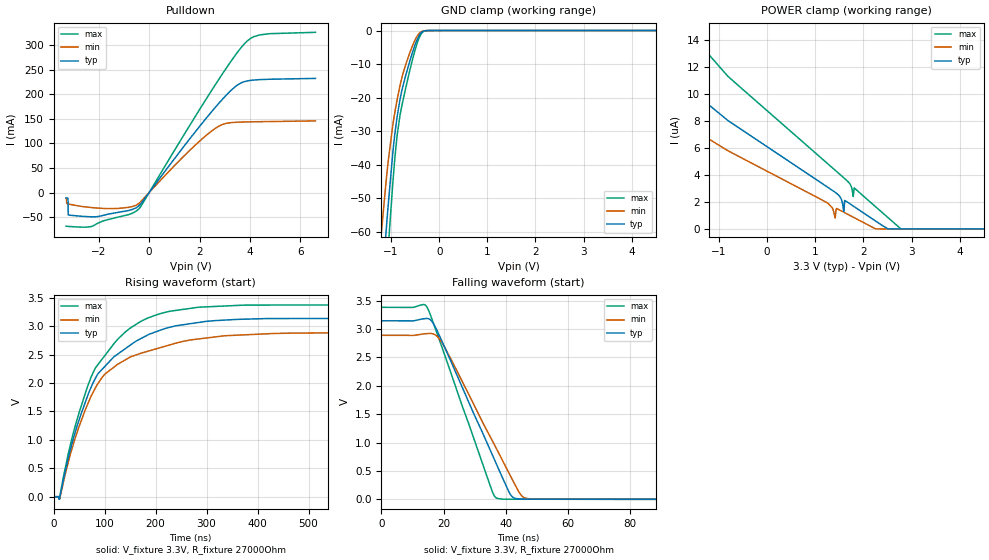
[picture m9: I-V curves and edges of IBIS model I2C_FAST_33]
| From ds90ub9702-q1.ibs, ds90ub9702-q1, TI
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|   I2C_Fast_33 Model
[Model]   I2C_FAST_33
Model_type   I/O_open_drain
Polarity   Non-Inverting
Enable   Active-High
Vinl = 0.99
Vinh = 2.31
Vmeas = 1.65
Vref = 3.3
Cref = 0pF
Rref = 27000
|   typ   min   max
C_comp   1.392003pF   1.392003pF   1.392003pF
[Voltage Range]   3.3   3   3.6
[Temperature Range]   27   105   -40
[Pullup Reference]   3.3   3   3.6
[Pulldown Reference]   -0   0   -0
[Power Clamp Reference]   3.3   3   3.6
[GND Clamp Reference]   0   0   0
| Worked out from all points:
|   slope of the pulldown table from 0 to 0.495 V, typ, clamps not added: 14.5 ohm
|   GND clamp passes 1 mA (typ) near -0.39 V on its own axis
|   falling waveform, V_fixture 3.3V, R_fixture 27000Ohm: 20-80 % time 15.3ns typ, 16.1ns min, 12.9ns max; typ from 3.14 V to 0.002 V
|   rising waveform, V_fixture 3.3V, R_fixture 27000Ohm: 20-80 % time 99.2ns typ, 94.8ns min, 92.5ns max; typ from 0.002 V to 3.14 V
[Pulldown]
|   Voltage   I(typ)   I(min)   I(max)
-3.3V     -10.66mA   -11.81mA   -68.45mA
-3.27V    -10.84mA   -22.15mA   -68.58mA
-3.221V   -11.73mA   -23.04mA   -68.79mA
-3.211V   -45.65mA   -23.2mA    -68.83mA
-2.32V    -49.24mA   -30.33mA   -69.34mA
-1.241V   -40.33mA   -32.32mA   -49.99mA
-419.1mV  -27.53mA   -22.53mA   -33.72mA
2.511V    166.3mA    126.3mA    210.1mA
3.343V    212.1mA    142.6mA    273.8mA
3.907V    227.1mA    143.7mA    308.7mA
4.402V    229.7mA    144.1mA    320.7mA
6.6V      232.1mA    145.7mA    325.8mA
[GND Clamp]
|   Voltage   I(typ)   I(min)   I(max)
-3.3V     -528.6mA   -466.9mA   -595.9mA
-1.211V   -80.34mA   -61.77mA   -97.81mA
-1.102V   -59.67mA   -44.82mA   -73.84mA
-1.063V   -52.53mA   -39.35mA   -65.39mA
-943.8mV  -33.69mA   -26.31mA   -41.91mA
-874.5mV  -25.73mA   -20.64mA   -31.31mA
-815.1mV  -20.61mA   -16.48mA   -25.31mA
-706.2mV  -13.96mA   -10.63mA   -17.82mA
-567.6mV  -7.079mA   -5.004mA   -9.374mA
-458.7mV  -2.703mA   -1.686mA   -3.845mA
-359.7mV  -460.5uA   -270uA     -723.2uA
6.6V      0A         0A         0A
[POWER Clamp]
|   Voltage   I(typ)   I(min)   I(max)
-3.3V     42.87uA    22.78uA    77.21uA
-2.993V   23.33uA    15.21uA    37.79uA
-2.488V   14.76uA    10.86uA    22.03uA
-1.419V   9.829uA    7.138uA    13.8uA
1.254V    3.108uA    1.927uA    4.861uA
1.412V    2.723uA    806.8nA    4.365uA
1.591V    1.287uA    1.246uA    3.805uA
1.61V     2.116uA    1.209uA    3.742uA
1.789V    1.703uA    874.7nA    2.413uA
1.808V    1.656uA    837.6nA    3.045uA
2.779V    0A         0A         7.004nA
6.6V      0A         0A         0A
[Ramp]
R_load = 27000
|   typ   min   max
dV/dt_r   1.88511/9.90096e-08   1.73155/9.48974e-08   2.02719/9.2589e-08
dV/dt_f   1.88528/1.52584e-08   1.7316/1.61125e-08   2.02734/1.29191e-08
[Falling Waveform]
V_fixture = 3.3V
V_fixture_min = 3V
V_fixture_max = 3.6V
R_fixture = 27000Ohm
C_fixture = 0F
|   Time   V(typ)   V(min)   V(max)
0s        3.144V     2.888V     3.38V
14.71ns   3.185V     2.918V     3.381V
16.41ns   3.12V      2.915V     3.149V
19.18ns   2.819V     2.783V     2.725V
35.8ns    771mV      1.022V     123.6mV
38.8ns    400.4mV    702.7mV    5.427mV
42.38ns   34.25mV    321.9mV    4.081mV
45.51ns   5.012mV    45.26mV    3.829mV
49.21ns   4.691mV    6.654mV    3.53mV
1.25us    1.787mV    2.013mV    1.579mV
[Rising Waveform]
V_fixture = 3.3V
V_fixture_min = 3V
V_fixture_max = 3.6V
R_fixture = 27000Ohm
C_fixture = 0F
|   Time   V(typ)   V(min)   V(max)
0s        1.787mV    2.013mV    1.579mV
11.21ns   -33.34mV   -5.142mV   -44.58mV
41.98ns   1.118V     1.017V     1.229V
81.17ns   2.067V     1.898V     2.25V
101.6ns   2.302V     2.163V     2.495V
142.3ns   2.615V     2.416V     2.91V
205.6ns   2.917V     2.612V     3.21V
299.3ns   3.084V     2.791V     3.339V
432.7ns   3.133V     2.871V     3.371V
1.25us    3.144V     2.888V     3.38V
